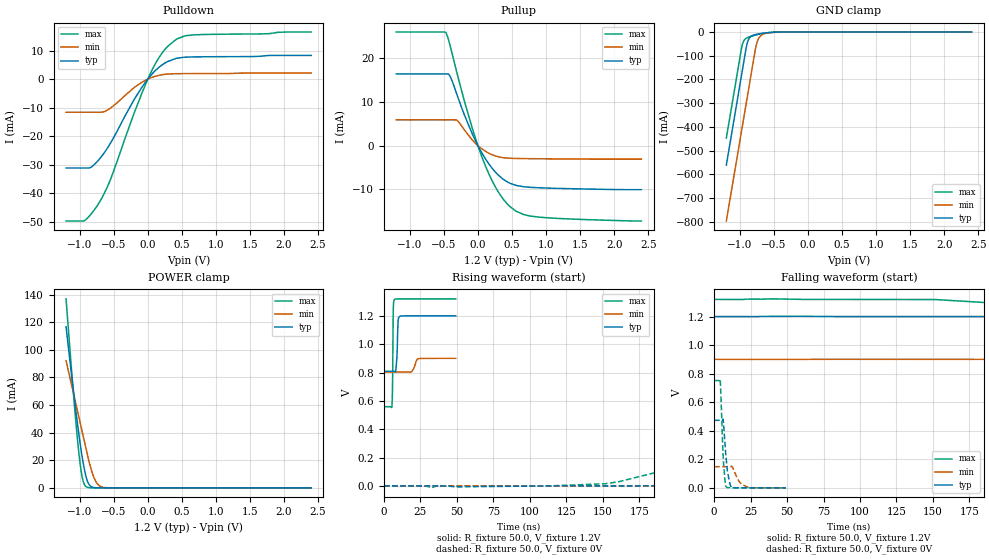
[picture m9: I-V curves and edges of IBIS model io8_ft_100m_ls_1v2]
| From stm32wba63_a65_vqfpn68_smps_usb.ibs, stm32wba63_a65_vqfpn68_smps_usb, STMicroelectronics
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[Model]   io8_ft_100m_ls_1v2
Model_type I/O
Polarity   Non-Inverting
Enable   Active-Low
| CAP_THRESHOLD on pad IOFT is "UDTCAPC" :
| Rising=30.0% of vddiom   Falling=70.0% of vddiom
| C_comp min and max val. don't necessarily correlate with the min and max pvt
| but are the smallest and greatest pad capacitance found.
| var   typ   min   max
C_comp   2.88584pF  2.81061pF  2.98919pF
|C_comp_pullup   1.64681pF  1.48756pF  1.78716pF
|C_comp_pulldown   1.23903pF  1.32305pF  1.20203pF
Vinl = 450.0mV
Vinh = 660.0mV
Vmeas = 600.0mV   | Reference voltage for timing measurements
Cref  = 50.0pF   | Timing specification test load capacitance value
Rref  = 1.0MOhm   | Timing specification test load resistance value
Vref  = 660.0mV   | Timing specification test load voltage
[Model Spec]
| TIME_THRESHOLD on pin ZIV11 is "CMOS" :
| Rising=50.0% of vdd   Falling=50.0% of vdd
Vinl 441.50000mV 335.50000mV 487.50000mV
Vinh 755.50000mV 552.50000mV 839.50000mV
| variable   typ   min   max
[Temperature Range] 25.0 140.0 -40.0
| variable   typ   min   max
[Voltage Range] 1.2V 900.0mV 1.32V
| variable   typ   min   max
[POWER Clamp Reference] 1.2V 900.0mV 1.32V
| variable   typ   min   max
[GND Clamp Reference] 0V 0V 0V
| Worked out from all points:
|   slope of the pulldown table from 0 to 0.18 V, typ, clamps not added: 40.6 ohm
|   slope of the pullup table from 0 to 0.18 V, typ, clamps not added: 39.4 ohm
|   GND clamp passes 1 mA (typ) near -0.51 V on its own axis
|   POWER clamp passes 1 mA (typ) near -0.83 V on its own axis
|   rising waveform, R_fixture 50.0, V_fixture 1.2V: 20-80 % time 789ps typ, 2.05ns min, 412ps max; typ from 0.809 V to 1.2 V
|   falling waveform, R_fixture 50.0, V_fixture 1.2V: 20-80 % time 303ns typ, 752ns min, 158ns max; typ from 1.2 V to 0.809 V
|   rising waveform, R_fixture 50.0, V_fixture 0V: 20-80 % time 349ns typ, 851ns min, 185ns max; typ from 0 V to 0.473 V
|   falling waveform, R_fixture 50.0, V_fixture 0V: 20-80 % time 2.54ns typ, 4.81ns min, 1.84ns max; typ from 0.473 V to 0 V
[POWER Clamp]
-1.2V     116.7mA    92.13mA    136.9mA
-1.09V    69.42mA    68.21mA    67.14mA
-1.02V    41.75mA    52.99mA    28.91mA
-990mV    30.98mA    46.47mA    16.09mA
-970mV    24.36mA    42.12mA    9.575mA
-940mV    15.59mA    35.6mA     3.485mA
-910mV    8.693mA    29.07mA    1.01mA
-860mV    2.259mA    18.59mA    104.6uA
-780mV    143.1uA    6.246mA    2.555uA
-720mV    16.22uA    1.846mA    157.1nA
-650mV    1.267uA    330.3uA    6.118nA
2.4V      0A         0A         0A
[GND Clamp]
-1.2V     -561.6mA   -797.4mA   -447.4mA
-980mV    -187.6mA   -423.4mA   -73.43mA
-960mV    -153.6mA   -389.4mA   -48.26mA
-900mV    -54.17mA   -287.4mA   -24.97mA
-870mV    -29.55mA   -236.4mA   -21.19mA
-830mV    -17.05mA   -168.4mA   -17.42mA
-760mV    -9.921mA   -54.55mA   -11.89mA
-730mV    -8.191mA   -29.78mA   -9.811mA
-690mV    -6.26mA    -14.49mA   -7.318mA
-600mV    -2.976mA   -4.315mA   -3.058mA
-380mV    -57.63uA   -251uA     -19.49uA
2.4V      872.8pA    204.8nA    349.4pA
| variable   typ   min   max
[Pullup Reference] 1.2V 900.0mV 1.32V
| variable   typ   min   max
[Pulldown Reference] 0V 0V 0V
[Pullup]
-1.2V     16.39mA    5.903mA    25.96mA
-470mV    16.39mA    5.903mA    25.8mA
-410mV    15.89mA    5.903mA    22.96mA
-310mV    11.76mA    5.823mA    16.75mA
-80mV     2.58mA     1.232mA    3.849mA
80mV      -2.237mA   -962.6uA   -3.434mA
190mV     -4.777mA   -1.94mA    -7.418mA
310mV     -6.857mA   -2.571mA   -10.82mA
540mV     -8.979mA   -2.91mA    -14.76mA
670mV     -9.371mA   -2.949mA   -15.71mA
920mV     -9.627mA   -2.991mA   -16.35mA
2.4V      -10.04mA   -3.075mA   -17.21mA
[Pulldown]
-1.2V     -31.2mA    -11.62mA   -49.78mA
-930mV    -31.2mA    -11.62mA   -49.64mA
-830mV    -30.86mA   -11.62mA   -47.25mA
-710mV    -28.04mA   -11.62mA   -43.19mA
-550mV    -22.55mA   -10.2mA    -35.3mA
-200mV    -7.146mA   -2.964mA   -11.89mA
40mV      1.171mA    405.8uA    2.092mA
130mV     3.416mA    1.118mA    6.182mA
230mV     5.302mA    1.613mA    9.763mA
420mV     7.288mA    1.898mA    13.99mA
670mV     7.779mA    1.924mA    15.51mA
2.4V      8.312mA    2.101mA    16.51mA
[Ramp]
dV/dt_r 283.79508mV/67.25732ns 88.93239mV/167.56948ns 450.99277mV/37.01515ns
dV/dt_f 234.65963mV/57.86868ns 57.89324mV/147.78959ns 456.7358mV/31.4692ns
R_load = 50.0
| Removed startup time: 0s 0s 0s  .
| Removed end time: 49.2ns.
[Rising Waveform]
R_fixture   = 50.0
V_fixture   = 1.2V
V_fixture_min = 900.0mV
V_fixture_max = 1.32V
0s        808.9mV    803.5mV    558.8mV
5.45ns    808.9mV    803.5mV    560.7mV
5.9ns     808.9mV    803.5mV    723.8mV
6.4ns     809mV      803.5mV    1.24V
7.05ns    808.5mV    803.5mV    1.314V
8.85ns    900.8mV    803.5mV    1.319V
9.55ns    1.129V     803.5mV    1.319V
10.05ns   1.189V     803.5mV    1.319V
24.1ns    1.2V       898.2mV    1.32V
49.2ns    1.2V       899.9mV    1.32V
| Removed startup time: 0s 0s 0s  .
| Removed end time: 9.996us.
[Falling Waveform]
R_fixture   = 50.0
V_fixture   = 1.2V
V_fixture_min = 900.0mV
V_fixture_max = 1.32V
0s        1.2V       900mV      1.32V
198.5ns   1.2V       900.1mV    1.286V
242.8ns   1.2V       900mV      1.182V
347.8ns   1.178V     900mV      813.5mV
442.3ns   1.104V     900mV      669.3mV
612ns     937mV      899.9mV    588.4mV
816ns     857.8mV    898.1mV    565.9mV
1.224us   817.2mV    870.2mV    559.2mV
2.61us    808.9mV    808.6mV    558.8mV
9.996us   808.9mV    803.5mV    558.8mV
| Removed startup time: 0s 0s 0s  .
| Removed end time: 9.996us.
[Rising Waveform]
R_fixture   = 50.0
V_fixture   = 0V
V_fixture_min = 0V
V_fixture_max = 0V
0s        4.648nV    215.3nV    3.229nV
156.7ns   -86.22uV   -29.46uV   22.38mV
333.5ns   54.83mV    -11.28uV   496.5mV
408ns     132.3mV    18.11uV    621.7mV
504ns     232.6mV    114.5uV    700.2mV
660.3ns   352.8mV    612.7uV    739.9mV
816ns     417.7mV    4.156mV    748.7mV
1.143us   462.6mV    35.58mV    751.4mV
2.652us   472.9mV    141.7mV    751.6mV
9.996us   473mV      148.2mV    751.7mV
| Removed startup time: 0s 0s 0s  .
| Removed end time: 49.2ns.
[Falling Waveform]
R_fixture   = 50.0
V_fixture   = 0V
V_fixture_min = 0V
V_fixture_max = 0V
0s        473mV      148.3mV    751.7mV
4.2ns     473mV      148.3mV    755.8mV
6.25ns    476.1mV    148.3mV    217.1mV
7.45ns    314.2mV    148.3mV    54.66mV
8.1ns     225.6mV    148.3mV    9.169mV
9.1ns     119.3mV    148.3mV    2.31mV
12.05ns   2.925mV    152.2mV    435.9uV
17.65ns   221.5uV    38.19mV    173.5uV
22.1ns    95.81uV    8.443mV    160.9uV
49.2ns    98.22uV    22.01uV    147.8uV
